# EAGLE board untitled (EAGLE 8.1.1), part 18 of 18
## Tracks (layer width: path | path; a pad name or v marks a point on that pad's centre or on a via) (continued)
S$18291 (continued)
  Bottom 0.381: 149.16,122.88 149.16,113.92
S$18292
  Bottom 0.381: 215.84,132.97 215.84,135.09
S$18293
  Bottom 0.381: 215.84,135.09 213.02,137.91
S$18294
  Bottom 0.381: 213.02,137.91 206.02,137.91
S$18295
  Bottom 0.381: 206.02,137.91 197.05,146.88
S$18296
  Bottom 0.381: 197.05,146.88 178.11,146.88
S$18297
  Bottom 0.381: 178.11,146.88 172.97,152.02
S$18298
  Bottom 0.381: 306.59,143.12 305.59,144.12
S$18299
  Bottom 0.381: 305.59,144.12 305.59,159.45
S$18300
  Bottom 0.381: 305.59,159.45 306.53,160.39
S$18301
  Bottom 0.381: 306.53,160.39 309.12,160.39
S$18302
  Bottom 0.381: 309.12,160.39 311.25,158.26
S$18303
  Bottom 0.381: 311.25,158.26 318.62,158.26
S$18304
  Bottom 0.381: 318.62,158.26 319.33,158.97
S$18305
  Bottom 0.381: 319.33,158.97 319.33,170.55
S$18306
  Bottom 0.381: 319.33,170.55 319.84,171.05
S$18307
  Bottom 0.381: 70.27,108.61 70.27,104.08
S$18308
  Bottom 0.381: 70.27,104.08 61.06,94.87
S$18309
  Bottom 0.381: 44.39,132.97 50.99,126.36
S$18310
  Bottom 0.381: 50.99,126.36 65.66,126.36
S$18311
  Bottom 0.381: 65.66,126.36 69.14,122.88
S$18312
  Bottom 0.381: 69.14,122.88 69.14,120.71
S$18313
  Bottom 0.381: 69.14,120.71 71.61,118.23
S$18314
  Bottom 0.381: 71.61,118.23 71.61,115.39
S$18315
  Bottom 0.381: 71.61,115.39 70.27,114.05
S$18316
  Bottom 0.381: 70.27,114.05 70.27,108.61
S$18317
  Bottom 0.381: 197.76,158.6 223.95,132.41
S$18318
  Bottom 0.381: 223.95,132.41 232.59,132.41
S$18319
  Bottom 0.381: 232.59,132.41 233.54,131.46
S$18320
  Bottom 0.381: 233.54,131.46 235.53,131.46
S$18321
  Bottom 0.381: 235.53,131.46 242.3,138.22
S$18322
  Bottom 0.381: 242.3,138.22 242.3,138.72
S$18323
  Bottom 0.381: 64.39,158.6 63.52,157.73
S$18324
  Bottom 0.381: 63.52,157.73 46.2,157.73
S$18325
  Bottom 0.381: 46.2,157.73 45.34,158.6
S$18326
  Bottom 0.381: 102.49,158.6 102.05,158.16
S$18327
  Bottom 0.381: 102.05,158.16 83.89,158.16
S$18328
  Bottom 0.381: 83.89,158.16 83.44,158.6
S$18329
  Bottom 0.381: 140.6,158.6 140.25,158.26
S$18330
  Bottom 0.381: 140.25,158.26 121.89,158.26
S$18331
  Bottom 0.381: 121.89,158.26 121.55,158.6
S$18332
  Bottom 0.635: 303.2,107.34 303.2,120.03
S$18333
  Bottom 0.635: 303.2,120.03 301.6,121.63
S$18334
  Bottom 0.635: 301.6,121.63 301.6,124.79
S$18335
  Bottom 0.635: 44.39,143.84 44.39,143.87
S$18336
  Bottom 0.635: 44.39,143.87 45.85,145.33
S$18337
  Bottom 0.635: 45.85,145.33 61.96,145.33
S$18338
  Bottom 0.635: 61.96,145.33 63.44,143.84
S$18339
  Bottom 0.635: 68.2,165.27 68.57,165.64
S$18340
  Bottom 0.635: 68.57,165.64 74.99,165.64
S$18341
  Bottom 0.635: 74.99,165.64 77.73,162.89
S$18342
  Bottom 0.635: 11.88,139.09 1.28,128.49
S$18343
  Bottom 0.635: 1.28,128.49 1.28,103.59
S$18344
  Bottom 0.635: 16.26,139.09 11.88,139.09
S$18345
  Bottom 0.635: 11.88,139.09 11.73,139.25
S$18346
  Bottom 0.635: 11.73,139.25 11.73,150.58
S$18347
  Bottom 0.635: 11.73,150.58 15.81,154.66
S$18348
  Bottom 0.635: 15.81,154.66 15.81,162.89
S$18349
  Bottom 0.635: 163.47,165.27 170.62,165.27
S$18350
  Bottom 0.635: 170.62,165.27 172.99,162.89
S$18351
  Bottom 0.635: 249.2,162.89 251.11,162.89
S$18352
  Bottom 0.635: 251.11,162.89 253.49,160.51
S$18353
  Bottom 0.635: 301.6,162.89 301.6,165.27
S$18354
  Bottom 0.635: 320.64,162.89 320.64,165.27
S$18355
  Bottom 0.635: 182.52,165.27 189.67,165.27
S$18356
  Bottom 0.635: 189.67,165.27 192.04,162.89
S$18357
  Bottom 0.635: 172.99,162.89 180.15,162.89
S$18358
  Bottom 0.635: 180.15,162.89 182.52,165.27
S$18359
  Bottom 0.635: 15.81,162.89 13.42,162.89
S$18360
  Bottom 0.635: 13.42,162.89 11.05,165.27
S$18361
  Bottom 0.635: 17,143.84 17.19,143.66
S$18362
  Bottom 0.635: 17.19,143.66 17.19,140.02
S$18363
  Bottom 0.635: 17.19,140.02 16.26,139.09
S$18364
  Bottom 0.635: 17,127.17 19.94,130.1
S$18365
  Bottom 0.635: 19.94,130.1 19.94,135.41
S$18366
  Bottom 0.635: 19.94,135.41 16.26,139.09
S$18367
  Bottom 0.635: 168.23,124.79 167.94,124.79
S$18368
  Bottom 0.635: 167.94,124.79 160.45,132.28
S$18369
  Bottom 0.635: 177.66,122.92 170.1,122.92
S$18370
  Bottom 0.635: 170.1,122.92 168.23,124.79
S$18371
  Bottom 0.635: 160.45,132.28 152.96,124.79
S$18372
  Bottom 0.635: 152.96,124.79 149.17,124.79
S$18373
  Bottom 0.635: 158.7,143.84 160.45,142.09
S$18374
  Bottom 0.635: 160.45,142.09 160.45,132.28
S$18375
  Bottom 0.635: 61.06,105.74 61.06,102.97
S$18376
  Bottom 0.635: 61.06,102.97 58.24,100.15
S$18377
  Bottom 0.635: 58.24,100.15 42.84,100.15
S$18378
  Bottom 0.635: 42.84,100.15 41.77,101.21
S$18379
  Bottom 0.635: 53.92,124.79 58.17,120.53
S$18380
  Bottom 0.635: 58.17,120.53 58.17,108.63
S$18381
  Bottom 0.635: 58.17,108.63 61.06,105.74
S$18382
  Bottom 0.635: 265.87,143.84 270.64,143.84
S$18383
  Bottom 0.635: 270.64,143.84 277.54,150.75
S$18384
  Bottom 0.635: 82.49,143.84 82.49,135.41
S$18385
  Bottom 0.635: 82.49,135.41 78.91,131.82
S$18386
  Bottom 0.635: 78.91,131.82 78.66,131.82
S$18387
  Bottom 0.635: 125.36,165.2 132.57,165.2
S$18388
  Bottom 0.635: 132.57,165.2 134.89,162.89
S$18389
  Bottom 0.635: 115.83,162.89 123.05,162.89
S$18390
  Bottom 0.635: 123.05,162.89 125.36,165.2
S$18391
  Bottom 0.635: 125.36,165.2 125.36,165.27
S$18392
  Bottom 0.635: 78.66,131.82 66.65,143.84
S$18393
  Bottom 0.635: 66.65,143.84 63.44,143.84
S$18394
  Bottom 0.635: 72.97,124.79 78.66,130.49
S$18395
  Bottom 0.635: 78.66,130.49 78.66,131.82
S$18396
  Bottom 0.635: 39.63,162.89 37.25,165.27
S$18397
  Bottom 0.635: 37.25,165.27 30.1,165.27
S$18398
  Bottom 0.635: 49.15,165.27 46.78,162.89
S$18399
  Bottom 0.635: 46.78,162.89 39.63,162.89
S$18400
  Bottom 0.635: 229.91,120.26 227.77,118.12
S$18401
  Bottom 0.635: 227.77,118.12 227.77,105.74
S$18402
  Bottom 0.635: 225.38,124.79 229.91,120.27
S$18403
  Bottom 0.635: 229.91,120.27 229.91,120.26
S$18404
  Bottom 0.635: 58.68,162.9 56.31,165.27
S$18405
  Bottom 0.635: 56.31,165.27 49.15,165.27
S$18406
  Bottom 0.635: 87.26,165.27 84.88,162.89
S$18407
  Bottom 0.635: 84.88,162.89 77.73,162.89
S$18408
  Bottom 0.635: 96.78,162.89 94.4,165.27
S$18409
  Bottom 0.635: 94.4,165.27 87.26,165.27
S$18410
  Bottom 0.635: 301.6,105.74 303.2,107.34
S$18411
  Bottom 0.635: 303.2,107.34 319.04,107.34
S$18412
  Bottom 0.635: 319.04,107.34 320.64,105.74
S$18413
  Bottom 0.635: 103.78,162.89 96.78,162.89
S$18414
  Bottom 0.635: 206.33,124.79 206.33,116.72
S$18415
  Bottom 0.635: 206.33,116.72 203.95,114.33
S$18416
  Bottom 0.635: 203.95,114.33 203.95,105.74
S$18417
  Bottom 0.635: 195.17,142.2 206.33,131.04
S$18418
  Bottom 0.635: 206.33,131.04 206.33,124.79
S$18419
  Bottom 0.635: 106.31,165.27 103.94,162.89
S$18420
  Bottom 0.635: 103.94,162.89 103.78,162.89
S$18421
  Bottom 0.635: 101.55,143.84 103.78,146.07
S$18422
  Bottom 0.635: 103.78,146.07 103.78,162.89
S$18423
  Bottom 0.635: 103.18,142.2 101.55,143.84
S$18424
  Bottom 0.635: 195.17,142.2 196.81,143.84
S$18425
  Bottom 0.635: 179.39,142.2 195.17,142.2
S$18426
  Bottom 0.635: 95.51,124.5 103.18,132.17
S$18427
  Bottom 0.635: 103.18,132.17 103.18,142.2
S$18428
  Bottom 0.635: 103.18,142.2 118.96,142.2
S$18429
  Bottom 0.635: 118.96,142.2 120.6,143.84
S$18430
  Bottom 0.635: 179.39,142.2 177.76,143.84
S$18431
  Bottom 0.635: 178.09,123.15 178.09,126.45
S$18432
  Bottom 0.635: 178.09,126.45 179.39,127.75
S$18433
  Bottom 0.635: 179.39,127.75 179.39,142.2
S$18434
  Bottom 0.635: 95.51,124.5 95.22,124.79
S$18435
  Bottom 0.635: 95.22,124.79 92.02,124.79
S$18436
  Bottom 0.635: 107.16,112.86 95.51,124.5
S$18437
  Bottom 0.635: 177.66,122.92 177.86,122.92
S$18438
  Bottom 0.635: 177.86,122.92 178.09,123.15
S$18439
  Bottom 0.635: 178.09,123.15 185.64,123.15
S$18440
  Bottom 0.635: 185.64,123.15 187.28,124.8
S$18441
  Bottom 0.635: 272.54,117.88 272.54,116.17
S$18442
  Bottom 0.635: 273.81,117.88 273.81,116.17
S$18443
  Bottom 0.635: 275.08,117.88 275.08,116.17
S$18444
  Bottom 0.635: 276.35,117.88 276.35,116.17
S$18445
  Bottom 0.635: 276.35,116.17 277.26,115.26
S$18446
  Bottom 0.635: 277.26,115.26 277.26,111.02
S$18447
  Bottom 0.635: 277.26,111.02 282.54,105.73
S$18448
  Bottom 0.635: 276.35,116.17 275.08,116.17
S$18449
  Bottom 0.635: 273.81,116.17 272.54,116.17
S$18450
  Bottom 0.635: 275.08,116.17 273.81,116.17
S$18451
  Bottom 0.635: 111.07,124.8 111.07,116.57
S$18452
  Bottom 0.635: 111.07,116.57 107.36,112.86
S$18453
  Bottom 0.635: 107.36,112.86 107.16,112.86
S$18454
  Bottom 0.635: 106.29,97.29 107.16,98.15
S$18455
  Bottom 0.635: 107.16,98.15 107.16,112.86
S$18456
  Bottom 0.635: 177.66,97.36 177.66,122.92
S$18457
  Bottom 0.381: 145.36,139.55 145.09,139.29
S$18458
  Bottom 0.381: 145.09,139.29 126.57,139.29
S$18459
  Bottom 0.381: 126.57,139.29 126.31,139.55
S$18460
  Bottom 0.381: 240.62,139.55 240.32,139.24
S$18461
  Bottom 0.381: 240.32,139.24 221.88,139.24
S$18462
  Bottom 0.381: 221.88,139.24 221.57,139.55
S$18463
  Bottom 0.381: 298.97,127.88 300.76,126.1
S$18464
  Bottom 0.381: 300.76,126.1 302.14,126.1
S$18465
  Bottom 0.381: 302.14,126.1 304.08,124.15
S$18466
  Bottom 0.381: 304.08,124.15 304.08,120.46
S$18467
  Bottom 0.381: 258.49,95.73 259.71,96.95
S$18468
  Bottom 0.381: 259.71,96.95 259.71,113.04
S$18469
  Bottom 0.381: 259.71,113.04 259.49,113.26
S$18470
  Bottom 0.381: 259.49,113.26 259.49,114.7
S$18471
  Bottom 0.381: 259.49,114.7 260.55,115.76
S$18472
  Bottom 0.381: 260.55,115.76 260.55,117.49
S$18473
  Bottom 0.381: 113.93,105.73 115.26,105.73
S$18474
  Bottom 0.381: 115.26,105.73 117.11,107.59
S$18475
  Bottom 0.381: 44.15,101.45 43.08,102.52
S$18476
  Bottom 0.381: 43.08,102.52 36.7,102.52
S$18477
  Bottom 0.381: 36.7,102.52 34.08,99.9
S$18478
  Bottom 0.381: 34.08,99.9 29.46,99.9
S$18479
  Bottom 0.381: 29.46,99.9 22.2,92.64
S$18480
  Bottom 0.381: 22.2,92.64 17.48,92.64
S$18481
  Bottom 0.381: 185.38,105.73 185.38,114.3
S$18482
  Bottom 0.381: 185.38,114.3 191.57,120.5
S$18483
  Bottom 0.381: 191.57,120.5 192.99,120.5
S$18484
  Bottom 0.381: 291.35,127.88 292.94,126.29
S$18485
  Bottom 0.381: 292.94,126.29 296.09,126.29
S$18486
  Bottom 0.381: 296.09,126.29 299.37,123.02
S$18487
  Bottom 0.381: 307.31,158.6 308.9,157
S$18488
  Bottom 0.381: 308.9,157 308.9,150.87
S$18489
  Bottom 0.381: 308.9,150.87 315.59,144.18
S$18490
  Bottom 0.381: 315.59,144.18 315.59,136.88
S$18491
  Bottom 0.381: 315.59,136.88 306.59,127.88
S$18492
  Bottom 0.381: 69.16,139.55 68.84,139.24
S$18493
  Bottom 0.381: 68.84,139.24 50.41,139.24
S$18494
  Bottom 0.381: 50.41,139.24 50.1,139.55
S$18495
  Bottom 0.381: 189.43,177.66 187.13,179.95
S$18496
  Bottom 0.381: 187.13,179.95 80.72,179.95
S$18497
  Bottom 0.381: 80.72,179.95 59.07,158.29
S$18498
  Bottom 0.381: 59.07,158.29 52.61,158.29
S$18499
  Bottom 0.381: 52.61,158.29 51.18,159.73
S$18500
  Bottom 0.381: 51.18,159.73 39.13,159.73
S$18501
  Bottom 0.381: 39.13,159.73 37.66,158.26
S$18502
  Bottom 0.381: 37.66,158.26 26.63,158.26
S$18503
  Bottom 0.381: 26.63,158.26 26.29,158.6
S$18504
  Bottom 0.381: 311.67,127.88 316.15,132.36
S$18505
  Bottom 0.381: 316.15,132.36 316.15,150.55
S$18506
  Bottom 0.381: 316.15,150.55 309.46,157.24
S$18507
  Bottom 0.381: 309.46,157.24 309.46,158.28
S$18508
  Bottom 0.381: 309.46,158.28 307.91,159.84
S$18509
  Bottom 0.381: 307.91,159.84 306.76,159.84
S$18510
  Bottom 0.381: 306.76,159.84 306.15,159.22
S$18511
  Bottom 0.381: 306.15,159.22 306.15,157.31
S$18512
  Bottom 0.381: 306.15,157.31 306.39,157.07
S$18513
  Bottom 0.381: 244.2,177.66 244.01,177.66
S$18514
  Bottom 0.381: 244.01,177.66 238.07,171.72
S$18515
  Bottom 0.381: 238.07,171.72 238.07,169.19
S$18516
  Bottom 0.381: 238.07,169.19 245.36,161.9
S$18517
  Bottom 0.381: 245.36,161.9 245.36,158.98
S$18518
  Bottom 0.381: 245.36,158.98 246.17,158.18
S$18519
  Bottom 0.381: 246.17,158.18 248.53,158.18
S$18520
  Bottom 0.381: 248.53,158.18 253.88,152.83
S$18521
  Bottom 0.381: 287.07,170.51 285.94,169.38
S$18522
  Bottom 0.381: 285.94,169.38 285.94,155.22
S$18523
  Bottom 0.381: 285.94,155.22 284.95,154.24
S$18524
  Bottom 0.381: 281.1,120.28 281.1,129.73
S$18525
  Bottom 0.381: 281.1,129.73 290.56,139.19
S$18526
  Bottom 0.381: 290.56,139.19 290.56,138.68
S$18527
  Bottom 0.381: 314.21,127.88 316.85,130.51
S$18528
  Bottom 0.381: 316.85,130.51 316.85,151.17
S$18529
  Bottom 0.381: 316.85,151.17 322.17,156.5
S$18530
  Bottom 0.381: 322.17,156.5 322.17,171.62
S$18531
  Bottom 0.381: 322.17,171.62 317.37,176.42
S$18532
  Bottom 0.381: 296.47,178.67 300.19,174.95
S$18533
  Bottom 0.381: 300.19,174.95 300.19,172.62
S$18534
  Bottom 0.381: 300.19,172.62 299.27,171.7
S$18535
  Bottom 0.381: 299.27,171.7 299.27,169.84
S$18536
  Bottom 0.381: 299.27,169.84 300.27,168.83
S$18537
  Bottom 0.381: 300.27,168.83 300.27,159.08
S$18538
  Bottom 0.381: 300.27,159.08 299.44,158.24
S$18539
  Bottom 0.381: 299.44,158.24 294.75,158.24
S$18540
  Bottom 0.381: 294.75,158.24 292.62,160.37
S$18541
  Bottom 0.381: 292.62,160.37 292.62,163.92
S$18542
  Bottom 0.381: 292.62,163.92 293.98,165.27
S$18543
  Bottom 0.635: 265.68,178.69 266.25,178.69
S$18544
  Bottom 0.635: 266.25,178.69 275.87,169.06
S$18545
  Bottom 0.635: 275.87,169.06 275.87,166.66
S$18546
  Bottom 0.635: 317.3,178.67 317.3,178.05
S$18547
  Bottom 0.635: 317.3,178.05 316.23,176.99
S$18548
  Bottom 0.635: 316.23,176.99 315.77,176.99
S$18549
  Bottom 0.635: 315.77,176.99 313.4,174.62
S$18550
  Bottom 0.635: 313.4,174.62 313.4,172.59
S$18551
  Bottom 0.635: 313.4,172.59 318.06,167.94
S$18552
  Bottom 0.635: 318.06,167.94 318.06,159.62
S$18553
  Bottom 0.635: 299.01,178.67 300.39,180.06
S$18554
  Bottom 0.635: 300.39,180.06 316.56,180.06
S$18555
  Bottom 0.635: 316.56,180.06 317.3,179.32
S$18556
  Bottom 0.635: 317.3,179.32 317.3,178.67
S$18557
  Bottom 0.635: 146.62,121.54 146.62,131.06
S$18558
  Bottom 0.635: 146.62,131.06 156.15,140.59
S$18559
  Bottom 0.635: 160.91,178.69 162.17,177.43
S$18560
  Bottom 0.635: 162.17,177.43 162.17,172.56
S$18561
  Bottom 0.635: 162.17,172.56 161.68,172.07
S$18562
  Bottom 0.635: 161.68,172.07 161.68,163.21
S$18563
  Bottom 0.635: 161.68,163.21 166.64,158.25
S$18564
  Bottom 0.635: 166.64,158.25 169.05,158.25
S$18565
  Bottom 0.635: 169.05,158.25 170.43,159.64
S$18566
  Bottom 0.635: 199.01,178.69 200.27,177.43
S$18567
  Bottom 0.635: 200.27,177.43 200.27,172.56
S$18568
  Bottom 0.635: 200.27,172.56 199.85,172.15
S$18569
  Bottom 0.635: 199.85,172.15 199.85,170.34
S$18570
  Bottom 0.635: 199.85,170.34 208.53,161.66
S$18571
  Bottom 0.635: 208.53,161.66 208.53,159.64
S$18572
  Bottom 0.635: 146.36,154.62 141.07,159.91
S$18573
  Bottom 0.635: 141.07,159.91 132.6,159.91
S$18574
  Bottom 0.635: 132.6,159.91 132.33,159.64
S$18575
  Bottom 0.635: 146.36,154.62 151.38,159.64
S$18576
  Bottom 0.635: 137.1,140.59 137.1,145.35
S$18577
  Bottom 0.635: 137.1,145.35 146.36,154.62
S$18578
  Bottom 0.635: 218.06,178.69 219.32,177.43
S$18579
  Bottom 0.635: 219.32,177.43 219.32,172.56
S$18580
  Bottom 0.635: 219.32,172.56 218.9,172.15
S$18581
  Bottom 0.635: 218.9,172.15 218.9,170.43
S$18582
  Bottom 0.635: 218.9,170.43 227.58,161.75
S$18583
  Bottom 0.635: 227.58,161.75 227.58,159.64
S$18584
  Bottom 0.635: 8.51,178.69 9.77,177.43
S$18585
  Bottom 0.635: 9.77,177.43 9.77,172.56
S$18586
  Bottom 0.635: 9.77,172.56 9.41,172.2
S$18587
  Bottom 0.635: 9.41,172.2 9.41,164.16
S$18588
  Bottom 0.635: 9.41,164.16 13.27,160.3
S$18589
  Bottom 0.635: 13.27,160.3 13.27,159.64
S$18590
  Bottom 0.635: 90.99,132.76 89.47,131.24
S$18591
  Bottom 0.635: 89.47,131.24 89.47,121.54
S$18592
  Bottom 0.635: 90.99,132.76 86.43,137.32
S$18593
  Bottom 0.635: 86.43,137.32 86.43,139.07
S$18594
  Bottom 0.635: 99,140.59 91.17,132.76
S$18595
  Bottom 0.635: 91.17,132.76 90.99,132.76
S$18596
  Bottom 0.635: 20.42,121.54 26.67,115.29
S$18597
  Bottom 0.635: 26.67,115.29 34.7,107.25
S$18598
  Bottom 0.635: 26.67,115.29 13.87,102.49
S$18599
  Bottom 0.635: 13.87,102.49 10.89,102.49
S$18600
  Bottom 0.635: 55.68,107.25 34.7,107.25
S$18601
  Bottom 0.635: 58.52,102.49 55.68,105.33
S$18602
  Bottom 0.635: 55.68,105.33 55.68,107.25
S$18603
  Bottom 0.635: 51.37,121.54 55.68,117.23
S$18604
  Bottom 0.635: 55.68,117.23 55.68,107.25
S$18605
  Bottom 0.635: 34.7,107.25 34.7,102.49
S$18606
  Bottom 0.635: 169.98,117.23 173.18,117.23
S$18607
  Bottom 0.635: 173.18,117.23 176.64,120.69
S$18608
  Bottom 0.635: 169.98,117.23 165.67,121.54
S$18609
  Bottom 0.635: 163.15,97.36 163.15,97.54
S$18610
  Bottom 0.635: 163.15,97.54 169.98,104.37
S$18611
  Bottom 0.635: 169.98,104.37 169.98,117.23
S$18612
  Bottom 0.635: 198.63,126.23 196.82,126.23
S$18613
  Bottom 0.635: 196.82,126.23 192.13,121.54
S$18614
  Bottom 0.635: 192.13,121.54 184.72,121.54
S$18615
  Bottom 0.635: 203.77,121.54 203.77,121.88
S$18616
  Bottom 0.635: 203.77,121.88 199.41,126.23
S$18617
  Bottom 0.635: 199.41,126.23 198.63,126.23
S$18618
  Bottom 0.635: 198.63,126.23 198.63,136.2
S$18619
  Bottom 0.635: 198.63,136.2 194.25,140.59
S$18620
  Bottom 0.635: 142.12,117.03 146.62,121.54
S$18621
  Bottom 0.635: 142.12,117.03 142.12,113.3
S$18622
  Bottom 0.635: 142.12,113.3 131.3,102.49
S$18623
  Bottom 0.635: 131.3,102.49 129.96,102.49
S$18624
  Bottom 0.635: 142.12,117.03 137.36,121.8
S$18625
  Bottom 0.635: 137.36,121.8 127.83,121.8
S$18626
  Bottom 0.635: 127.83,121.8 127.57,121.54
S$18627
  Bottom 0.635: 222.67,121.54 222.67,128.65
S$18628
  Bottom 0.635: 222.67,128.65 216.91,134.42
S$18629
  Bottom 0.635: 216.91,134.42 216.91,136.97
S$18630
  Bottom 0.635: 216.91,136.97 213.3,140.59
S$18631
  Bottom 0.635: 225.2,102.49 225.2,102.87
S$18632
  Bottom 0.635: 225.2,102.87 218.69,109.39
S$18633
  Bottom 0.635: 218.69,109.39 218.36,109.39
S$18634
  Bottom 0.635: 218.36,109.39 217.34,110.4
S$18635
  Bottom 0.635: 217.34,110.4 217.34,116.06
S$18636
  Bottom 0.635: 217.34,116.06 222.67,121.39
S$18637
  Bottom 0.635: 222.67,121.39 222.67,121.54
S$18638
  Bottom 0.635: 222.67,121.54 222.82,121.54
S$18639
  Bottom 0.635: 286.97,122.99 286.97,103.47
S$18640
  Bottom 0.635: 286.97,103.47 285.79,102.29
S$18641
  Bottom 0.635: 286.27,127.88 286.97,127.18
S$18642
  Bottom 0.635: 286.97,127.18 286.97,122.99
S$18643
  Bottom 0.635: 298.25,121.52 298.25,122.17
S$18644
  Bottom 0.635: 298.25,122.17 297.43,122.99
S$18645
  Bottom 0.635: 297.43,122.99 286.97,122.99
S$18646
  Bottom 0.635: 285.79,102.29 285.79,100.91
S$18647
  Bottom 0.635: 285.79,100.91 286.51,100.19
S$18648
  Bottom 0.635: 286.51,100.19 296.53,100.19
S$18649
  Bottom 0.635: 296.53,100.19 298.25,101.9
S$18650
  Bottom 0.635: 298.25,101.9 298.25,102.47
S$18651
  Bottom 0.635: 279.96,102.47 280.15,102.29
S$18652
  Bottom 0.635: 280.15,102.29 285.79,102.29
S$18653
  Bottom 0.635: 258.54,121.54 249.02,112.01
S$18654
  Bottom 0.635: 249.02,112.01 249.02,102.49
S$18655
  Bottom 0.635: 263.3,140.59 257.63,134.92
S$18656
  Bottom 0.635: 257.63,134.92 257.63,122.44
S$18657
  Bottom 0.635: 257.63,122.44 258.54,121.54
S$18658
  Bottom 0.635: 91.77,97.28 75.92,113.13
S$18659
  Bottom 0.635: 75.92,113.13 75.92,116.04
S$18660
  Bottom 0.635: 75.92,116.04 70.42,121.54
S$18661
  Bottom 0.635: 265.68,178.69 264.3,177.3
S$18662
  Bottom 0.635: 264.3,177.3 247.19,177.3
S$18663
  Bottom 0.635: 247.19,177.3 245.51,178.98
S$18664
  Bottom 0.635: 245.51,178.98 237.4,178.98
S$18665
  Bottom 0.635: 237.4,178.98 237.11,178.69
S$18666
  Bottom 0.635: 294.25,180.06 297.5,180.06
S$18667
  Bottom 0.635: 297.5,180.06 298.24,179.32
S$18668
  Bottom 0.635: 298.24,179.32 298.24,178.67
S$18669
  Bottom 0.635: 283.91,173.27 283.91,175.13
S$18670
  Bottom 0.635: 283.91,175.13 288.84,180.06
S$18671
  Bottom 0.635: 288.84,180.06 294.25,180.06
S$18672
  Bottom 0.635: 294.25,180.06 294.25,172.69
S$18673
  Bottom 0.635: 294.25,172.69 299.01,167.94
S$18674
  Bottom 0.635: 299.01,167.94 299.01,159.62
S$18675
  Bottom 0.635: 317.29,102.47 318.05,102.47
S$18676
  Bottom 0.635: 283.91,173.27 284.3,173.27
S$18677
  Bottom 0.635: 281.88,166.66 281.88,171.52
S$18678
  Bottom 0.635: 281.88,171.52 283.62,173.27
S$18679
  Bottom 0.635: 283.62,173.27 283.91,173.27
S$18680
  Bottom 0.635: 270.45,159.64 275.87,165.06
S$18681
  Bottom 0.635: 275.87,165.06 275.87,166.66
S$18682
  Bottom 0.635: 275.87,166.66 281.88,166.66
S$18683
  Bottom 0.635: 282.08,166.66 281.88,166.66
S$18684
  Bottom 0.635: 283.46,166.66 282.08,166.66
S$18685
  Bottom 0.381: 296.43,127.88 300.29,124.02
S$18686
  Bottom 0.381: 300.29,124.02 300.29,115.61
S$18687
  Bottom 0.381: 300.29,115.61 297.85,113.16
S$18688
  Bottom 0.381: 297.85,113.16 297.85,111.81
S$18689
  Bottom 0.381: 297.85,111.81 289.44,103.41
S$18690
  Bottom 0.381: 289.44,103.41 289.44,101.45
S$18691
  Bottom 0.381: 269.2,101.45 260.99,93.24
S$18692
  Bottom 0.381: 260.99,93.24 246.45,93.24
S$18693
  Bottom 0.381: 246.45,93.24 238.24,101.45
S$18694
  Bottom 0.381: 276.66,102.47 276.66,103.74
S$18695
  Bottom 0.381: 276.66,103.74 274.92,105.48
S$18696
  Bottom 0.381: 274.92,105.48 274.92,105.73
S$18697
  Bottom 0.381: 107.26,131.93 112.73,131.93
S$18698
  Bottom 0.381: 112.73,131.93 114.24,130.43
S$18699
  Bottom 0.381: 275.39,92.31 270.72,92.31
S$18700
  Bottom 0.381: 270.72,92.31 269.2,93.83
S$18701
  Bottom 0.381: 294.44,92.31 288.58,92.31
S$18702
  Bottom 0.381: 288.58,92.31 287.07,93.83
S$18703
  Bottom 0.381: 314.76,102.47 314.76,103.74
S$18704
  Bottom 0.381: 314.76,103.74 313.02,105.48
S$18705
  Bottom 0.381: 313.02,105.48 313.02,105.74
S$18706
  Bottom 0.381: 314.76,178.67 314.76,177.4
S$18707
  Bottom 0.381: 314.76,177.4 311.97,174.62
S$18708
  Bottom 0.381: 311.97,174.62 311.97,166.32
S$18709
  Bottom 0.381: 311.97,166.32 313.02,165.27
S$18710
  Bottom 0.381: 295.71,159.62 295.71,160.89
S$18711
  Bottom 0.381: 295.71,160.89 293.98,162.63
S$18712
  Bottom 0.381: 293.98,162.63 293.98,162.89
S$18713
  Bottom 0.381: 295.71,102.47 295.71,103.74
S$18714
  Bottom 0.381: 295.71,103.74 293.98,105.48
S$18715
  Bottom 0.381: 293.98,105.48 293.98,105.74
S$18716
  Bottom 0.381: 314.76,159.62 314.76,160.89
S$18717
  Bottom 0.381: 314.76,160.89 313.02,162.63
S$18718
  Bottom 0.381: 313.02,162.63 313.02,162.89
S$18719
  Bottom 0.381: 192.99,112.88 198.46,112.88
S$18720
  Bottom 0.381: 198.46,112.88 199.96,111.38
S$18721
  Bottom 0.381: 294.44,111.36 289.77,111.36
S$18722
  Bottom 0.381: 289.77,111.36 288.25,112.88
S$18723
  Bottom 0.381: 267.91,159.64 269.18,159.64
S$18724
  Bottom 0.381: 269.18,159.64 269.18,159.07
S$18725
  Bottom 0.381: 269.18,159.07 269.88,158.37
S$18726
  Bottom 0.381: 269.88,158.37 277.54,158.37
S$18727
  Bottom 0.381: 178.71,150.98 184.17,150.98
S$18728
  Bottom 0.381: 184.17,150.98 185.67,149.48
S$18729
  Bottom 0.381: 253.73,148.6 243.7,148.6
S$18730
  Bottom 0.381: 243.7,148.6 242.82,149.48
S$18731
  Bottom 0.381: 173.94,120.5 168.66,120.5
S$18732
  Bottom 0.381: 168.66,120.5 166.36,122.8
S$18733
  Bottom 0.381: 166.36,122.8 165.1,122.8
S$18734
  Bottom 0.381: 165.1,122.8 164.39,122.09
S$18735
  Bottom 0.381: 164.39,122.09 164.39,120.39
S$18736
  Bottom 0.381: 164.39,120.39 164.13,120.13
S$18737
  Bottom 0.381: 164.13,120.13 155.25,120.13
S$18738
  Bottom 0.381: 155.25,120.13 154.89,120.5
S$18739
  Bottom 0.381: 97.73,120.5 97.38,120.14
S$18740
  Bottom 0.381: 97.38,120.14 79.03,120.14
S$18741
  Bottom 0.381: 79.03,120.14 78.68,120.5
S$18742
  Bottom 0.381: 135.84,120.5 135.45,120.11
S$18743
  Bottom 0.381: 135.45,120.11 117.17,120.11
S$18744
  Bottom 0.381: 117.17,120.11 116.79,120.5
S$18745
  Bottom 0.381: 154.89,112.88 160.36,112.88
S$18746
  Bottom 0.381: 160.36,112.88 161.86,111.38
S$18747
  Bottom 0.381: 144.08,121.54 144.08,122.81
S$18748
  Bottom 0.381: 144.08,122.81 143.54,122.81
S$18749
  Bottom 0.381: 143.54,122.81 141.55,124.79
S$18750
  Bottom 0.381: 294.43,149.46 289.77,149.46
S$18751
  Bottom 0.381: 289.77,149.46 288.25,150.98
S$18752
  Bottom 0.381: 294.43,168.51 292.69,168.51
S$18753
  Bottom 0.381: 292.69,168.51 287.07,162.89
S$18754
  Bottom 0.381: 283.46,170.68 285.9,173.11
S$18755
  Bottom 0.381: 285.9,173.11 285.9,173.27
S$18756
  Bottom 0.381: 45.34,150.98 50.82,150.98
S$18757
  Bottom 0.381: 50.82,150.98 52.32,149.48
S$18758
  Bottom 0.381: 69.16,131.93 74.63,131.93
S$18759
  Bottom 0.381: 74.63,131.93 76.14,130.43
S$18760
  Bottom 0.381: 313.48,92.31 298.66,92.31
S$18761
  Bottom 0.381: 298.66,92.31 298.23,92.74
S$18762
  Bottom 0.381: 298.23,92.74 297.44,92.74
S$18763
  Bottom 0.381: 297.44,92.74 296.59,93.59
S$18764
  Bottom 0.381: 296.59,93.59 296.59,93.83
S$18765
  Bottom 0.381: 296.59,93.83 289.44,93.83
S$18766
  Bottom 0.381: 297.26,167.55 296.69,166.98
S$18767
  Bottom 0.381: 296.69,166.98 293.53,166.98
S$18768
  Bottom 0.381: 293.53,166.98 289.45,162.89
S$18769
  Bottom 0.381: 307.31,150.98 308.83,149.46
S$18770
  Bottom 0.381: 308.83,149.46 309.04,149.46
S$18771
  Bottom 0.381: 50.1,131.93 55.58,131.93
S$18772
  Bottom 0.381: 55.58,131.93 57.09,130.43
S$18773
  Bottom 0.381: 25.1,92.64 23.3,90.84
S$18774
  Bottom 0.381: 23.3,90.84 8.57,90.84
S$18775
  Bottom 0.381: 8.57,90.84 7.08,92.33
S$18776
  Bottom 0.381: 246.48,102.49 247.75,102.49
S$18777
  Bottom 0.381: 247.75,102.49 247.75,101.85
S$18778
  Bottom 0.381: 247.75,101.85 248.38,101.22
S$18779
  Bottom 0.381: 248.38,101.22 254.93,101.22
S$18780
  Bottom 0.381: 254.93,101.22 256.11,102.4
S$18781
  Bottom 0.381: 280.44,116.06 281.1,115.4
S$18782
  Bottom 0.381: 281.1,115.4 281.1,112.66
S$18783
  Bottom 0.381: 272.54,114.47 271.77,115.24
S$18784
  Bottom 0.381: 271.77,115.24 271.77,119.34
S$18785
  Bottom 0.381: 271.77,119.34 271.88,119.45
S$18786
  Bottom 0.381: 271.88,119.45 277.05,119.45
S$18787
  Bottom 0.381: 277.05,119.45 280.44,116.06
S$18788
  Bottom 0.381: 280.44,116.06 284.67,120.28
S$18789
  Bottom 0.381: 272.54,112.88 272.54,114.47
S$18790
  Bottom 0.381: 220.28,121.54 220.28,122.81
S$18791
  Bottom 0.381: 220.28,122.81 219.75,122.81
S$18792
  Bottom 0.381: 219.75,122.81 217.76,124.79
S$18793
  Bottom 0.381: 201.23,121.54 201.23,122.81
S$18794
  Bottom 0.381: 201.23,122.81 200.7,122.81
S$18795
  Bottom 0.381: 200.7,122.81 198.71,124.79
S$18796
  Bottom 0.381: 225.04,159.64 225.04,160.91
S$18797
  Bottom 0.381: 225.04,160.91 224.52,160.91
S$18798
  Bottom 0.381: 224.52,160.91 222.53,162.89
S$18799
  Bottom 0.381: 39.31,140.59 39.31,141.86
S$18800
  Bottom 0.381: 39.31,141.86 38.76,141.86
S$18801
  Bottom 0.381: 38.76,141.86 36.77,143.84
S$18802
  Bottom 0.381: 82.17,178.69 82.17,177.42
S$18803
  Bottom 0.381: 82.17,177.42 79.32,174.57
S$18804
  Bottom 0.381: 79.32,174.57 79.32,165.59
S$18805
  Bottom 0.381: 79.32,165.59 79.64,165.27
S$18806
  Bottom 0.381: 86.93,121.54 86.93,122.81
S$18807
  Bottom 0.381: 84.4,124.79 86.39,122.81
S$18808
  Bottom 0.381: 86.39,122.81 86.93,122.81
S$18809
  Bottom 0.381: 77.41,140.59 77.41,141.86
S$18810
  Bottom 0.381: 77.41,141.86 76.86,141.86
S$18811
  Bottom 0.381: 76.86,141.86 74.87,143.84
S$18812
  Bottom 0.381: 164.42,131.93 169.88,131.93
S$18813
  Bottom 0.381: 169.88,131.93 171.39,130.43
S$18814
  Bottom 0.381: 183.47,131.93 188.93,131.93
S$18815
  Bottom 0.381: 188.93,131.93 190.44,130.43
S$18816
  Bottom 0.381: 210.76,140.59 210.76,141.86
S$18817
  Bottom 0.381: 210.76,141.86 210.22,141.86
S$18818
  Bottom 0.381: 210.22,141.86 208.24,143.84
S$18819
  Bottom 0.381: 221.57,131.93 223.08,130.43
S$18820
  Bottom 0.381: 223.08,130.43 228.54,130.43
S$18821
  Bottom 0.381: 260.76,140.59 260.76,141.86
S$18822
  Bottom 0.381: 260.76,141.86 260.24,141.86
S$18823
  Bottom 0.381: 260.24,141.86 258.25,143.84
S$18824
  Bottom 0.381: 48.83,121.54 48.83,122.81
S$18825
  Bottom 0.381: 48.83,122.81 48.28,122.81
S$18826
  Bottom 0.381: 48.28,122.81 46.3,124.79
S$18827
  Bottom 0.381: 41.77,112.88 46.06,112.88
S$18828
  Bottom 0.381: 46.06,112.88 47.56,111.38
S$18829
  Bottom 0.381: 67.88,121.54 67.88,122.81
S$18830
  Bottom 0.381: 67.88,122.81 67.33,122.81
S$18831
  Bottom 0.381: 67.33,122.81 65.35,124.79
S$18832
  Bottom 0.381: 59.63,112.88 65.11,112.88
S$18833
  Bottom 0.381: 65.11,112.88 66.61,111.38
S$18834
  Bottom 0.381: 153.61,140.59 153.61,141.86
S$18835
  Bottom 0.381: 153.61,141.86 153.07,141.86
S$18836
  Bottom 0.381: 153.07,141.86 151.08,143.84
S$18837
  Bottom 0.381: 126.31,131.93 131.78,131.93
S$18838
  Bottom 0.381: 131.78,131.93 133.29,130.43
S$18839
  Bottom 0.381: 78.68,112.88 84.16,112.88
S$18840
  Bottom 0.381: 84.16,112.88 85.66,111.38
S$18841
  Bottom 0.381: 44.15,93.83 43.02,94.96
S$18842
  Bottom 0.381: 43.02,94.96 40.85,94.96
S$18843
  Bottom 0.381: 40.85,94.96 38.22,92.33
S$18844
  Bottom 0.381: 38.22,92.33 30.89,92.33
S$18845
  Bottom 0.381: 55.98,102.49 55.98,103.76
S$18846
  Bottom 0.381: 55.98,103.76 55.42,103.76
S$18847
  Bottom 0.381: 55.42,103.76 53.44,105.74
S$18848
  Bottom 0.381: 48.91,93.83 53.21,93.83
S$18849
  Bottom 0.381: 53.21,93.83 54.71,92.33
S$18850
  Bottom 0.381: 127.42,102.49 127.42,103.76
S$18851
  Bottom 0.381: 127.42,103.76 126.87,103.76
S$18852
  Bottom 0.381: 126.87,103.76 124.88,105.74
S$18853
  Bottom 0.381: 121.55,105.73 121.55,96.92
S$18854
  Bottom 0.381: 121.55,96.92 126.15,92.33
S$18855
  Bottom 0.381: 198.85,102.49 198.85,103.76
S$18856
  Bottom 0.381: 198.85,103.76 198.31,103.76
S$18857
  Bottom 0.381: 198.31,103.76 196.33,105.74
S$18858
  Bottom 0.381: 193,105.73 193,96.91
S$18859
  Bottom 0.381: 193,96.91 197.58,92.33
S$18860
  Bottom 0.381: 222.66,102.49 222.66,103.76
S$18861
  Bottom 0.381: 222.66,103.76 222.13,103.76
S$18862
  Bottom 0.381: 222.13,103.76 220.15,105.74
S$18863
  Bottom 0.381: 238.24,93.83 243.71,93.83
S$18864
  Bottom 0.381: 243.71,93.83 245.21,92.33
S$18865
  Bottom 0.381: 5.97,178.69 5.97,177.42
S$18866
  Bottom 0.381: 5.97,177.42 3.12,174.56
S$18867
  Bottom 0.381: 3.12,174.56 3.12,165.57
S$18868
  Bottom 0.381: 3.12,165.57 3.43,165.27
S$18869
  Bottom 0.381: 22.48,165.27 22.05,165.71
S$18870
  Bottom 0.381: 22.05,165.71 22.05,166.08
S$18871
  Bottom 0.381: 22.05,166.08 21.49,166.64
S$18872
  Bottom 0.381: 21.49,166.64 21.49,170.57
S$18873
  Bottom 0.381: 21.49,170.57 21.81,170.9
S$18874
  Bottom 0.381: 21.81,170.9 22.05,170.9
S$18875
  Bottom 0.381: 22.05,170.9 22.05,174.44
S$18876
  Bottom 0.381: 22.05,174.44 25.02,177.42
S$18877
  Bottom 0.381: 25.02,178.69 25.02,177.42
S$18878
  Bottom 0.381: 44.07,178.69 44.07,177.42
S$18879
  Bottom 0.381: 44.07,177.42 41.22,174.57
S$18880
  Bottom 0.381: 41.22,174.57 41.22,165.58
S$18881
  Bottom 0.381: 41.22,165.58 41.53,165.27
S$18882
  Bottom 0.381: 63.12,178.69 63.12,177.42
S$18883
  Bottom 0.381: 63.12,177.42 60.27,174.57
S$18884
  Bottom 0.381: 60.27,174.57 60.27,165.58
S$18885
  Bottom 0.381: 60.27,165.58 60.58,165.27
S$18886
  Bottom 0.381: 101.22,178.69 101.22,177.42
S$18887
  Bottom 0.381: 101.22,177.42 98.19,174.39
S$18888
  Bottom 0.381: 98.19,174.39 98.19,165.76
S$18889
  Bottom 0.381: 98.19,165.76 98.69,165.27
S$18890
  Bottom 0.381: 120.27,178.69 120.27,177.42
S$18891
  Bottom 0.381: 120.27,177.42 117.43,174.58
S$18892
  Bottom 0.381: 117.43,174.58 117.43,165.58
S$18893
  Bottom 0.381: 117.43,165.58 117.74,165.27
S$18894
  Bottom 0.381: 139.32,178.69 139.32,177.42
S$18895
  Bottom 0.381: 139.32,177.42 136.36,174.46
S$18896
  Bottom 0.381: 136.36,174.46 136.36,165.7
S$18897
  Bottom 0.381: 136.36,165.7 136.79,165.27
S$18898
  Bottom 0.381: 158.37,178.69 158.37,177.42
S$18899
  Bottom 0.381: 158.37,177.42 155.46,174.51
S$18900
  Bottom 0.381: 155.46,174.51 155.46,165.66
S$18901
  Bottom 0.381: 155.46,165.66 155.85,165.27
S$18902
  Bottom 0.381: 177.42,178.69 177.42,177.42
S$18903
  Bottom 0.381: 177.42,177.42 174.62,174.62
S$18904
  Bottom 0.381: 174.62,174.62 174.62,165.55
S$18905
  Bottom 0.381: 174.62,165.55 174.9,165.27
S$18906
  Bottom 0.381: 196.47,178.69 196.47,177.42
S$18907
  Bottom 0.381: 196.47,177.42 193.56,174.5
S$18908
  Bottom 0.381: 193.56,174.5 193.56,165.66
S$18909
  Bottom 0.381: 193.56,165.66 193.95,165.27
S$18910
  Bottom 0.381: 215.52,178.69 215.52,177.42
S$18911
  Bottom 0.381: 215.52,177.42 212.68,174.58
S$18912
  Bottom 0.381: 212.68,174.58 212.68,165.58
S$18913
  Bottom 0.381: 212.68,165.58 213,165.27
S$18914
  Bottom 0.381: 234.57,178.69 234.57,177.42
S$18915
  Bottom 0.381: 234.57,177.42 231.73,174.58
S$18916
  Bottom 0.381: 231.73,174.58 231.73,165.59
S$18917
  Bottom 0.381: 231.73,165.59 232.05,165.27
S$18918
  Bottom 0.381: 266.41,177.22 266.88,176.75
S$18919
  Bottom 0.381: 266.88,176.75 266.88,172.54
S$18920
  Bottom 0.381: 266.88,172.54 264.38,170.04
S$18921
  Bottom 0.381: 264.38,170.04 264.38,163.78
S$18922
  Bottom 0.381: 264.38,163.78 261.11,160.51
S$18923
  Bottom 0.381: 257.29,158.12 257.29,163.95
S$18924
  Bottom 0.381: 257.29,163.95 261.87,168.53
S$18925
  Bottom 0.381: 10.73,159.64 10.73,160.91
S$18926
  Bottom 0.381: 10.73,160.91 10.18,160.91
S$18927
  Bottom 0.381: 10.18,160.91 8.19,162.89
S$18928
  Bottom 0.381: 34.54,159.64 34.54,160.91
S$18929
  Bottom 0.381: 34.54,160.91 33.99,160.91
S$18930
  Bottom 0.381: 33.99,160.91 32.01,162.89
S$18931
  Bottom 0.381: 26.29,150.99 31.77,150.99
S$18932
  Bottom 0.381: 31.77,150.99 33.27,149.48
S$18933
  Bottom 0.381: 53.59,159.64 53.59,160.91
S$18934
  Bottom 0.381: 53.59,160.91 53.05,160.91
S$18935
  Bottom 0.381: 53.05,160.91 51.06,162.9
S$18936
  Bottom 0.381: 91.69,159.64 91.69,160.91
S$18937
  Bottom 0.381: 91.69,160.91 91.15,160.91
S$18938
  Bottom 0.381: 91.15,160.91 89.16,162.89
S$18939
  Bottom 0.381: 110.74,159.64 110.74,160.91
S$18940
  Bottom 0.381: 110.74,160.91 110.21,160.91
S$18941
  Bottom 0.381: 110.21,160.91 108.21,162.89
S$18942
  Bottom 0.381: 129.79,159.64 129.79,160.91
S$18943
  Bottom 0.381: 129.79,160.91 129.26,160.91
S$18944
  Bottom 0.381: 129.26,160.91 127.27,162.89
S$18945
  Bottom 0.381: 148.84,159.64 148.84,160.91
S$18946
  Bottom 0.381: 148.84,160.91 148.31,160.91
S$18947
  Bottom 0.381: 148.31,160.91 146.32,162.89
S$18948
  Bottom 0.381: 244.09,159.64 244.09,160.91
S$18949
  Bottom 0.381: 244.09,160.91 243.57,160.91
S$18950
  Bottom 0.381: 243.57,160.91 241.58,162.89
S$18951
  Bottom 0.381: 58.36,140.59 58.36,141.86
S$18952
  Bottom 0.381: 58.36,141.86 57.81,141.86
S$18953
  Bottom 0.381: 57.81,141.86 55.82,143.84
S$18954
  Bottom 0.381: 258.49,103.35 258.49,107.62
S$18955
  Bottom 0.381: 258.49,107.62 254.73,111.38
S$18956
  Bottom 0.381: 223.77,149.48 222.27,150.98
S$18957
  Bottom 0.381: 222.27,150.98 216.81,150.98
S$18958
  Bottom 0.381: 125.03,121.54 125.03,122.81
S$18959
  Bottom 0.381: 125.03,122.81 124.49,122.81
S$18960
  Bottom 0.381: 124.49,122.81 122.5,124.79
S$18961
  Bottom 0.381: 163.13,121.54 163.13,122.81
S$18962
  Bottom 0.381: 163.13,122.81 162.59,122.81
S$18963
  Bottom 0.381: 162.59,122.81 160.61,124.79
S$18964
  Bottom 0.381: 229.91,112.64 232.72,112.64
S$18965
  Bottom 0.381: 232.72,112.64 241.61,121.54
S$18966
  Bottom 0.381: 189.43,170.03 187.92,168.53
S$18967
  Bottom 0.381: 187.92,168.53 176.15,168.53
S$18968
  Bottom 0.381: 64.39,150.98 69.87,150.98
S$18969
  Bottom 0.381: 69.87,150.98 71.37,149.48
S$18970
  Bottom 0.381: 205.99,159.64 205.99,160.91
S$18971
  Bottom 0.381: 205.99,160.91 205.46,160.91
S$18972
  Bottom 0.381: 205.46,160.91 203.47,162.89
S$18973
  Bottom 0.381: 72.64,159.64 72.64,160.91
S$18974
  Bottom 0.381: 72.64,160.91 72.1,160.91
S$18975
  Bottom 0.381: 72.1,160.91 70.11,162.89
S$18976
  Bottom 0.381: 134.56,140.59 134.56,141.86
S$18977
  Bottom 0.381: 134.56,141.86 134.02,141.86
S$18978
  Bottom 0.381: 134.02,141.86 132.03,143.84
S$18979
  Bottom 0.381: 172.66,140.59 172.66,141.86
S$18980
  Bottom 0.381: 172.66,141.86 172.12,141.86
S$18981
  Bottom 0.381: 172.12,141.86 170.14,143.84
S$18982
  Bottom 0.381: 96.46,140.59 96.46,141.86
S$18983
  Bottom 0.381: 96.46,141.86 95.91,141.86
S$18984
  Bottom 0.381: 95.91,141.86 93.93,143.84
S$18985
  Bottom 0.381: 105.98,121.54 105.98,122.81
S$18986
  Bottom 0.381: 105.98,122.81 105.44,122.81
S$18987
  Bottom 0.381: 105.44,122.81 103.45,124.8
S$18988
  Bottom 0.381: 97.73,112.88 103.21,112.88
S$18989
  Bottom 0.381: 103.21,112.88 104.71,111.38
S$18990
  Bottom 0.381: 8.35,102.49 7.08,102.49
S$18991
  Bottom 0.381: 7.08,102.49 7.08,101.77
S$18992
  Bottom 0.381: 7.08,101.77 1.28,95.97
S$18993
  Bottom 0.381: 37.01,170.03 35.86,171.19
S$18994
  Bottom 0.381: 35.86,171.19 33.83,171.19
S$18995
  Bottom 0.381: 33.83,171.19 31.17,168.53
S$18996
  Bottom 0.381: 31.17,168.53 23.75,168.53
S$18997
  Bottom 0.381: 167.89,159.64 167.89,160.91
S$18998
  Bottom 0.381: 167.89,160.91 167.36,160.91
S$18999
  Bottom 0.381: 167.36,160.91 165.37,162.89
S$19000
  Bottom 0.381: 186.94,159.64 186.94,160.91
S$19001
  Bottom 0.381: 186.94,160.91 186.41,160.91
S$19002
  Bottom 0.381: 186.41,160.91 184.42,162.89
S$19003
  Bottom 0.381: 197.76,150.98 203.22,150.98
S$19004
  Bottom 0.381: 203.22,150.98 204.72,149.48
S$19005
  Bottom 0.381: 226.34,170.03 226.34,172.36
S$19006
  Bottom 0.381: 226.34,172.36 218.62,180.07
S$19007
  Bottom 0.381: 218.62,180.07 217.66,180.07
S$19008
  Bottom 0.381: 217.66,180.07 216.78,179.18
S$19009
  Bottom 0.381: 216.78,179.18 216.78,177.64
S$19010
  Bottom 0.381: 216.78,177.64 214.25,175.11
S$19011
  Bottom 0.381: 214.25,175.11 214.25,168.53
S$19012
  Bottom 0.635: 27.49,136.36 33.44,130.41
S$19013
  Bottom 0.635: 33.44,130.41 33.71,130.41
S$19014
  Bottom 0.635: 33.71,130.41 45.13,118.99
S$19015
  Bottom 0.203: 321.27,144.15 322.56,143.77
S$19016
  Bottom 0.203: 321.27,143.4 322.56,143.77
S$19017
  Bottom 0.203: 321.27,143.4 322.56,143.04
S$19018
  Bottom 0.203: 321.27,142.67 322.56,143.04
S$19019
  Bottom 0.203: 321.27,142.06 322.56,141.69
S$19020
  Bottom 0.203: 321.27,141.32 322.56,141.69
S$19021
  Bottom 0.203: 321.27,141.32 322.56,140.95
S$19022
  Bottom 0.203: 321.27,140.58 322.56,140.95
S$19023
  Bottom 0.203: 321.27,139.97 322.56,139.6
S$19024
  Bottom 0.203: 321.27,139.23 322.56,139.6
S$19025
  Bottom 0.203: 321.27,139.23 322.56,138.86
S$19026
  Bottom 0.203: 321.27,138.49 322.56,138.86
S$19027
  Bottom 0.203: 322.1,137.79 322.19,137.88
S$19028
  Bottom 0.203: 322.19,137.88 322.28,137.79
S$19029
  Bottom 0.203: 322.28,137.79 322.19,137.7
S$19030
  Bottom 0.203: 322.19,137.7 322.1,137.79
S$19031
  Bottom 0.203: 320.89,135.98 320.71,136.07
S$19032
  Bottom 0.203: 320.71,136.07 320.62,136.35
S$19033
  Bottom 0.203: 320.62,136.35 320.62,136.53
S$19034
  Bottom 0.203: 320.62,136.53 320.71,136.81
S$19035
  Bottom 0.203: 320.71,136.81 320.99,137
S$19036
  Bottom 0.203: 320.99,137 321.45,137.09
S$19037
  Bottom 0.203: 321.45,137.09 321.91,137.09
S$19038
  Bottom 0.203: 321.91,137.09 322.28,137
S$19039
  Bottom 0.203: 322.28,137 322.47,136.81
S$19040
  Bottom 0.203: 322.47,136.81 322.56,136.53
S$19041
  Bottom 0.203: 322.56,136.53 322.56,136.44
S$19042
  Bottom 0.203: 322.56,136.44 322.47,136.16
S$19043
  Bottom 0.203: 322.47,136.16 322.28,135.98
S$19044
  Bottom 0.203: 322.28,135.98 322,135.89
S$19045
  Bottom 0.203: 322,135.89 321.91,135.89
S$19046
  Bottom 0.203: 321.91,135.89 321.63,135.98
S$19047
  Bottom 0.203: 321.63,135.98 321.45,136.16
S$19048
  Bottom 0.203: 321.45,136.16 321.36,136.44
S$19049
  Bottom 0.203: 321.36,136.44 321.36,136.53
S$19050
  Bottom 0.203: 321.36,136.53 321.45,136.81
S$19051
  Bottom 0.203: 321.45,136.81 321.63,137
S$19052
  Bottom 0.203: 321.63,137 321.91,137.09
S$19053
  Bottom 0.203: 320.62,134.72 320.71,135
S$19054
  Bottom 0.203: 320.71,135 320.99,135.18
S$19055
  Bottom 0.203: 320.99,135.18 321.45,135.28
S$19056
  Bottom 0.203: 321.45,135.28 321.73,135.28
S$19057
  Bottom 0.203: 321.73,135.28 322.19,135.18
S$19058
  Bottom 0.203: 322.19,135.18 322.47,135
S$19059
  Bottom 0.203: 322.47,135 322.56,134.72
S$19060
  Bottom 0.203: 322.56,134.72 322.56,134.54
S$19061
  Bottom 0.203: 322.56,134.54 322.47,134.26
S$19062
  Bottom 0.203: 322.47,134.26 322.19,134.08
S$19063
  Bottom 0.203: 322.19,134.08 321.73,133.99
S$19064
  Bottom 0.203: 321.73,133.99 321.45,133.99
S$19065
  Bottom 0.203: 321.45,133.99 320.99,134.08
S$19066
  Bottom 0.203: 320.99,134.08 320.71,134.26
S$19067
  Bottom 0.203: 320.71,134.26 320.62,134.54
S$19068
  Bottom 0.203: 320.62,134.54 320.62,134.72
S$19069
  Bottom 0.203: 321.27,133.38 323.2,133.38
S$19070
  Bottom 0.203: 321.54,133.38 321.36,133.19
S$19071
  Bottom 0.203: 321.36,133.19 321.27,133
S$19072
  Bottom 0.203: 321.27,133 321.27,132.72
S$19073
  Bottom 0.203: 321.27,132.72 321.36,132.54
S$19074
  Bottom 0.203: 321.36,132.54 321.54,132.36
S$19075
  Bottom 0.203: 321.54,132.36 321.82,132.26
S$19076
  Bottom 0.203: 321.82,132.26 322,132.26
S$19077
  Bottom 0.203: 322,132.26 322.28,132.36
S$19078
  Bottom 0.203: 322.28,132.36 322.47,132.54
S$19079
  Bottom 0.203: 322.47,132.54 322.56,132.72
S$19080
  Bottom 0.203: 322.56,132.72 322.56,133
S$19081
  Bottom 0.203: 322.56,133 322.47,133.19
S$19082
  Bottom 0.203: 322.47,133.19 322.28,133.38
S$19083
  Bottom 0.203: 321.82,131.65 321.82,130.55
S$19084
  Bottom 0.203: 321.82,130.55 321.63,130.55
S$19085
  Bottom 0.203: 321.63,130.55 321.45,130.64
S$19086
  Bottom 0.203: 321.45,130.64 321.36,130.73
S$19087
  Bottom 0.203: 321.36,130.73 321.27,130.92
S$19088
  Bottom 0.203: 321.27,130.92 321.27,131.19
S$19089
  Bottom 0.203: 321.27,131.19 321.36,131.38
S$19090
  Bottom 0.203: 321.36,131.38 321.54,131.56
S$19091
  Bottom 0.203: 321.54,131.56 321.82,131.65
S$19092
  Bottom 0.203: 321.82,131.65 322,131.65
S$19093
  Bottom 0.203: 322,131.65 322.28,131.56
S$19094
  Bottom 0.203: 322.28,131.56 322.47,131.38
S$19095
  Bottom 0.203: 322.47,131.38 322.56,131.19
S$19096
  Bottom 0.203: 322.56,131.19 322.56,130.92
S$19097
  Bottom 0.203: 322.56,130.92 322.47,130.73
S$19098
  Bottom 0.203: 322.47,130.73 322.28,130.55
S$19099
  Bottom 0.203: 321.27,129.94 322.56,129.94
S$19100
  Bottom 0.203: 321.82,129.94 321.54,129.85
S$19101
  Bottom 0.203: 321.54,129.85 321.36,129.66
S$19102
  Bottom 0.203: 321.36,129.66 321.27,129.48
S$19103
  Bottom 0.203: 321.27,129.48 321.27,129.2
S$19104
  Bottom 0.203: 321.54,127.48 321.36,127.67
S$19105
  Bottom 0.203: 321.36,127.67 321.27,127.85
S$19106
  Bottom 0.203: 321.27,127.85 321.27,128.13
S$19107
  Bottom 0.203: 321.27,128.13 321.36,128.31
S$19108
  Bottom 0.203: 321.36,128.31 321.54,128.5
S$19109
  Bottom 0.203: 321.54,128.5 321.82,128.59
S$19110
  Bottom 0.203: 321.82,128.59 322,128.59
S$19111
  Bottom 0.203: 322,128.59 322.28,128.5
S$19112
  Bottom 0.203: 322.28,128.5 322.47,128.31
S$19113
  Bottom 0.203: 322.47,128.31 322.56,128.13
S$19114
  Bottom 0.203: 322.56,128.13 322.56,127.85
S$19115
  Bottom 0.203: 322.56,127.85 322.47,127.67
S$19116
  Bottom 0.203: 322.47,127.67 322.28,127.48
S$19117
  Bottom 0.203: 321.82,126.87 321.82,125.76
S$19118
  Bottom 0.203: 321.82,125.76 321.63,125.76
S$19119
  Bottom 0.203: 321.63,125.76 321.45,125.86
S$19120
  Bottom 0.203: 321.45,125.86 321.36,125.95
S$19121
  Bottom 0.203: 321.36,125.95 321.27,126.13
S$19122
  Bottom 0.203: 321.27,126.13 321.27,126.41
S$19123
  Bottom 0.203: 321.27,126.41 321.36,126.6
S$19124
  Bottom 0.203: 321.36,126.6 321.54,126.78
S$19125
  Bottom 0.203: 321.54,126.78 321.82,126.87
S$19126
  Bottom 0.203: 321.82,126.87 322,126.87
S$19127
  Bottom 0.203: 322,126.87 322.28,126.78
S$19128
  Bottom 0.203: 322.28,126.78 322.47,126.6
S$19129
  Bottom 0.203: 322.47,126.6 322.56,126.41
S$19130
  Bottom 0.203: 322.56,126.41 322.56,126.13
S$19131
  Bottom 0.203: 322.56,126.13 322.47,125.95
S$19132
  Bottom 0.203: 322.47,125.95 322.28,125.76
S$19133
  Bottom 0.203: 321.27,125.15 322.56,125.15
S$19134
  Bottom 0.203: 321.63,125.15 321.36,124.88
S$19135
  Bottom 0.203: 321.36,124.88 321.27,124.69
S$19136
  Bottom 0.203: 321.27,124.69 321.27,124.41
S$19137
  Bottom 0.203: 321.27,124.41 321.36,124.23
S$19138
  Bottom 0.203: 321.36,124.23 321.63,124.14
S$19139
  Bottom 0.203: 321.63,124.14 322.56,124.14
S$19140
  Bottom 0.203: 320.62,123.25 322.19,123.25
S$19141
  Bottom 0.203: 322.19,123.25 322.47,123.16
S$19142
  Bottom 0.203: 322.47,123.16 322.56,122.97
S$19143
  Bottom 0.203: 322.56,122.97 322.56,122.79
S$19144
  Bottom 0.203: 321.27,123.53 321.27,122.88
S$19145
  Bottom 0.203: 322.1,122.09 322.19,122.18
S$19146
  Bottom 0.203: 322.19,122.18 322.28,122.09
S$19147
  Bottom 0.203: 322.28,122.09 322.19,122
S$19148
  Bottom 0.203: 322.19,122 322.1,122.09
S$19149
  Bottom 0.203: 321.54,120.28 321.36,120.46
S$19150
  Bottom 0.203: 321.36,120.46 321.27,120.65
S$19151
  Bottom 0.203: 321.27,120.65 321.27,120.92
S$19152
  Bottom 0.203: 321.27,120.92 321.36,121.11
S$19153
  Bottom 0.203: 321.36,121.11 321.54,121.29
S$19154
  Bottom 0.203: 321.54,121.29 321.82,121.39
S$19155
  Bottom 0.203: 321.82,121.39 322,121.39
S$19156
  Bottom 0.203: 322,121.39 322.28,121.29
S$19157
  Bottom 0.203: 322.28,121.29 322.47,121.11
S$19158
  Bottom 0.203: 322.47,121.11 322.56,120.92
S$19159
  Bottom 0.203: 322.56,120.92 322.56,120.65
S$19160
  Bottom 0.203: 322.56,120.65 322.47,120.46
S$19161
  Bottom 0.203: 322.47,120.46 322.28,120.28
S$19162
  Bottom 0.203: 320.62,119.67 322.56,119.67
S$19163
  Bottom 0.203: 321.27,119.06 322.19,119.06
S$19164
  Bottom 0.203: 322.19,119.06 322.47,118.97
S$19165
  Bottom 0.203: 322.47,118.97 322.56,118.78
S$19166
  Bottom 0.203: 322.56,118.78 322.56,118.5
S$19167
  Bottom 0.203: 322.56,118.5 322.47,118.32
S$19168
  Bottom 0.203: 322.47,118.32 322.19,118.04
S$19169
  Bottom 0.203: 321.27,118.04 322.56,118.04
S$19170
  Bottom 0.203: 320.62,117.43 322.56,117.43
S$19171
  Bottom 0.203: 321.54,117.43 321.36,117.25
S$19172
  Bottom 0.203: 321.36,117.25 321.27,117.06
S$19173
  Bottom 0.203: 321.27,117.06 321.27,116.79
S$19174
  Bottom 0.203: 321.27,116.79 321.36,116.6
S$19175
  Bottom 0.203: 321.36,116.6 321.54,116.42
S$19176
  Bottom 0.203: 321.54,116.42 321.82,116.32
S$19177
  Bottom 0.203: 321.82,116.32 322,116.32
S$19178
  Bottom 0.203: 322,116.32 322.28,116.42
S$19179
  Bottom 0.203: 322.28,116.42 322.47,116.6
S$19180
  Bottom 0.203: 322.47,116.6 322.56,116.79
S$19181
  Bottom 0.203: 322.56,116.79 322.56,117.06
S$19182
  Bottom 0.203: 322.56,117.06 322.47,117.25
S$19183
  Bottom 0.203: 322.47,117.25 322.28,117.43
(copper drawn outside any net)
  shapes: Bottom area x172, Bottom circle x1242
